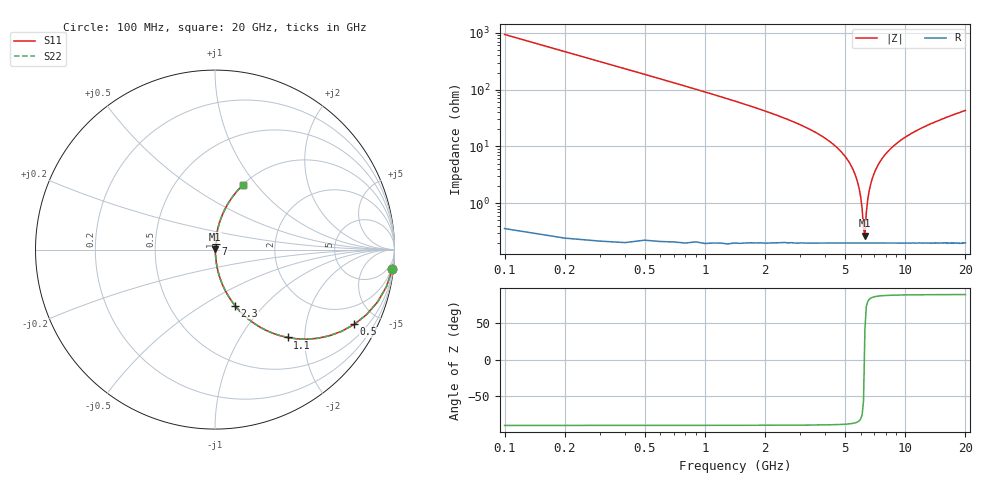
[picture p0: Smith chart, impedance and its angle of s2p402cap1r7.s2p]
! AVX Thin Film Operation		Date: April 2003
! Description: Accu-P® Series, Thin Film, SMD, RF Capacitor
! Part Number: 04023J1R7ABW
! 50 MHz  -  20 GHz
! Serial Measurements
# hz S db R 50
!	S11		S21		S12		S22
!	dB	Phase	dB	Phase	dB	Phase	dB	Phase
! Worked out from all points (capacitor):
!   200 points, 100 MHz to 20 GHz, reference 50 ohm
!   read as one part in series: C = 1.7 pF near 200 MHz
!   lowest |Z| = 270 mohm at 6.3 GHz (marker M1)
!   series resonance near 6.262 GHz, so ESL is about 380 pH
!   S11 on the Smith chart (normalised r, x): 100 MHz: 1, -19; 500 MHz: 1.00, -3.72; 1.1 GHz: 1.00, -1.65; 2.3 GHz: 1.00, -0.70; 7 GHz: 1.00, +0.07; 20 GHz: 1.00, +0.86
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1e8  -0.05 -6.1  -19.47 83.9  -19.47 83.9  -0.05 -6.1
2e8  -0.20 -12.1  -13.59 77.9  -13.59 77.9  -0.20 -12.1
3e8  -0.43 -17.8  -10.29 72.2  -10.29 72.2  -0.43 -17.8
5e8  -1.11 -28.2  -6.50 61.7  -6.50 61.7  -1.11 -28.2
1.1e9  -3.94 -50.4  -2.26 39.5  -2.26 39.5  -3.94 -50.4
2.3e9  -9.59 -70.3  -0.52 19.4  -0.52 19.4  -9.59 -70.3
3.5e9  -14.87 -79.0  -0.16 10.4  -0.16 10.4  -14.87 -79.0
4.8e9  -21.93 -84.0  -0.05 4.6  -0.05 4.6  -21.93 -84.0
5.6e9  -29.51 -84.7  -0.02 1.9  -0.02 1.9  -29.51 -84.7
6e9  -37.78 -80.4  -0.02 0.7  -0.02 0.7  -37.78 -80.4
6.1e9  -41.87 -75.2  -0.02 0.4  -0.02 0.4  -41.87 -75.2
6.2e9  -48.94 -55.9  -0.02 0.2  -0.02 0.2  -48.94 -55.9
6.3e9  -51.39 42.1  -0.02 -0.1  -0.02 -0.1  -51.39 42.1
6.4e9  -43.34 72.6  -0.02 -0.4  -0.02 -0.4  -43.34 72.6
6.5e9  -38.92 79.2  -0.02 -0.6  -0.02 -0.6  -38.92 79.2
6.8e9  -32.14 84.0  -0.02 -1.4  -0.02 -1.4  -32.14 84.0
7e9  -29.53 84.7  -0.02 -1.9  -0.02 -1.9  -29.53 84.7
8.1e9  -22.22 84.1  -0.04 -4.4  -0.04 -4.4  -22.22 84.1
1.01e10  -16.68 80.8  -0.11 -8.4  -0.11 -8.4  -16.68 80.8
1.34e10  -12.32 75.5  -0.28 -14.0  -0.28 -14.0  -12.32 75.5
1.67e10  -9.80 70.8  -0.50 -18.9  -0.50 -18.9  -9.80 70.8
2e10  -8.07 66.5  -0.75 -23.3  -0.75 -23.3  -8.07 66.5
